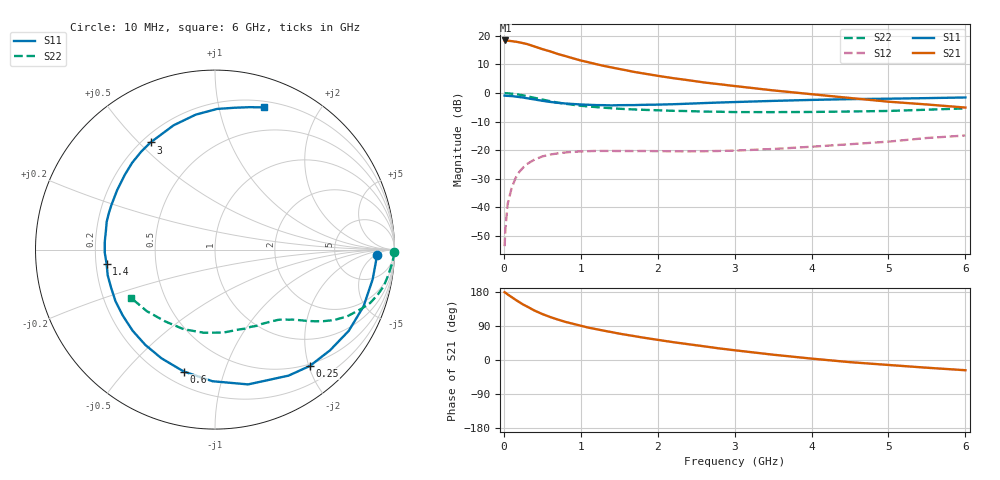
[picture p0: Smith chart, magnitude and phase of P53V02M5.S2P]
! SIEMENS Small Signal Semiconductors
! BFP183
! Si NPN RF Bipolar Junction Transistor in SOT143
! VCE = 3 V  IC = 2.5 mA
! Common Emitter S-Parameters:  March  1996
# GHz  S  MA  R  50
!  f  S11  S21  S12  S22
! GHz  MAG  ANG  MAG  ANG  MAG  ANG  MAG  ANG
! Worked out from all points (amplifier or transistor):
!   36 points, 10 MHz to 6 GHz, reference 50 ohm
!   highest |S21| = 18.4 dB at 20 MHz (marker M1)
!   |S21| within 3 dB of that: start of sweep to 496.5 MHz
!   unconditionally stable (mu >= 1): 1.982 GHz to 5.78 GHz
!   at 250 MHz: K = 0.13, MSG = 21.8 dB, |S12| = -26.1 dB
!   at 1.4 GHz: K = 0.74, MSG = 14.6 dB, |S12| = -20.2 dB
!   at 6 GHz: K = 0.96, MSG = 4.9 dB, |S12| = -14.8 dB
!   S11 on the Smith chart (normalised r, x): 10 MHz: 17, -6; 250 MHz: 0.47, -2.02; 600 MHz: 0.28, -0.74; 1.4 GHz: 0.24, -0.06; 3 GHz: 0.23, +0.54; 6 GHz: 0.26, +1.37
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0.01  0.9017 -2.0  8.285 178.8  0.0021 90.2  0.9987 -0.8
0.02  0.899 -4.3  8.328 177.8  0.0042 84.3  0.9976 -1.7
0.05  0.8939 -10.7  8.256 173.0  0.0115 86.6  0.9907 -4.1
0.15  0.8719 -31.3  7.937 159.3  0.0321 72.0  0.9624 -12.1
0.2  0.8518 -41.2  7.74 152.8  0.0417 67.4  0.9402 -15.6
0.25  0.8364 -50.8  7.462 146.5  0.0496 62.7  0.914 -19.0
0.3  0.8131 -59.7  7.217 141.3  0.0573 58.3  0.8822 -21.8
0.4  0.7734 -76.2  6.524 130.3  0.0689 49.8  0.8253 -26.8
0.5  0.7335 -91.1  5.874 121.3  0.0779 43.0  0.7711 -30.6
0.6  0.7012 -104.4  5.375 113.6  0.0841 37.9  0.7228 -33.5
0.7  0.6751 -116.2  4.837 106.8  0.0881 33.4  0.6822 -35.8
0.8  0.6577 -126.2  4.441 100.6  0.0914 29.8  0.65 -37.7
0.9  0.6442 -135.4  4.055 95.5  0.0942 26.9  0.6238 -39.2
1.1  0.6245 -152.6  3.461 85.4  0.0964 22.1  0.5826 -42.0
1.4  0.6091 -172.6  2.807 73.6  0.0972 17.7  0.5433 -46.0
1.8  0.6231 165.5  2.221 59.4  0.097 15.4  0.5102 -51.3
2.2  0.6382 148.6  1.824 47.1  0.0959 15.1  0.4897 -57.6
3  0.6968 121.0  1.329 25.7  0.0986 19.0  0.465 -73.1
3.5  0.73 108.4  1.115 14.0  0.1052 21.9  0.4646 -84.2
4.5  0.7837 89.2  0.821 -5.7  0.1275 24.7  0.4766 -111.4
5.5  0.8168 76.3  0.632 -20.4  0.1639 23.4  0.5119 -137.9
6  0.8378 71.0  0.558 -27.0  0.1812 19.9  0.5401 -150.3
